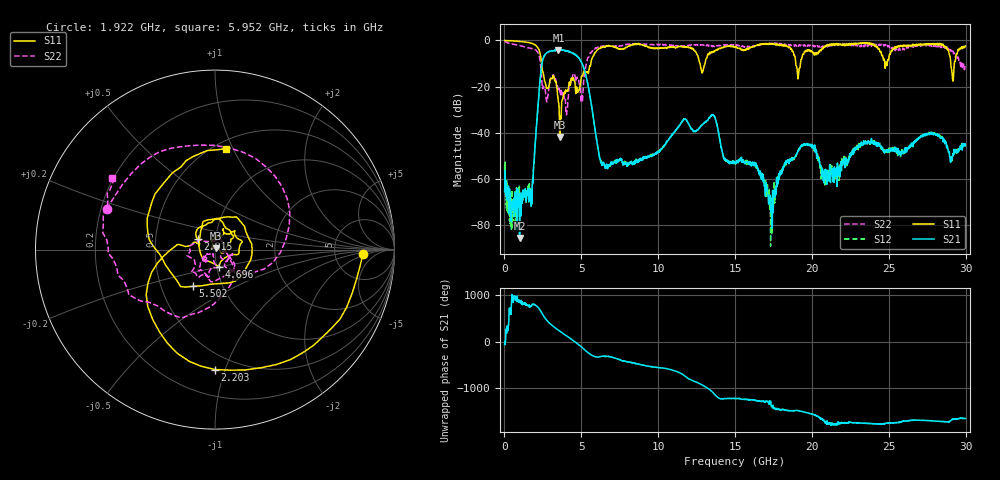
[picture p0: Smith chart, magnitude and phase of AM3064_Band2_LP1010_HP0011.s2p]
# Hz S DB R 50.0
!freq dBS11 angS11 dBS21 angS21 dBS12 angS12 dBS22 angS22
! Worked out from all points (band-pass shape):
!   1600 points, 10 MHz to 29.98 GHz, reference 50 ohm
!   highest |S21| = -4.09 dB at 3.515 GHz (marker M1); lowest = -85.6 dB at 984.7 MHz (marker M2)
!   |S21| within 3 dB of the highest: 2.559 GHz to 4.757 GHz (2.198 GHz wide, 60.1 % of centre)
!   lowest |S11| = -41.8 dB at 3.59 GHz (marker M3), VSWR 1.02, Z = 50.4 + j0.708 ohm
!   |S11| at or under -10 dB: 2.415 GHz to 5.619 GHz (3.205 GHz wide, 79.8 % of centre); 12.71 GHz to 13.05 GHz (330.9 MHz wide, 2.57 % of centre); 18.95 GHz to 19.25 GHz (304 MHz wide, 1.59 % of centre)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
!   |S22| runs from -32.2 to -0.3 dB; largest |S21 - S12| = 0.016
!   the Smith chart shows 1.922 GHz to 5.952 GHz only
!   S11 on the Smith chart (normalised r, x): 1.922 GHz: 10, -2; 2.203 GHz: 0.38, -0.92; 2.915 GHz: 0.82, +0.10; 4.696 GHz: 1.03, -0.20; 5.502 GHz: 0.72, -0.31; 5.952 GHz: 0.57, +0.94
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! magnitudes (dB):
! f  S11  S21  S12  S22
! 10 MHz  0.0  -65.5  -54.5  -0.3
! 328.6 MHz  -0.1  -64.3  -78.3  -1.3
! 984.7 MHz  -0.4  -85.6  -66.9  -2.2
! 1.922 GHz  -1.7  -52.5  -53.1  -3.8
! 2.203 GHz  -3.5  -26.4  -26.5  -5.5
! 2.915 GHz  -19.0  -4.8  -4.7  -19.1
! 3.515 GHz  -26.8  -4.1  -4.2  -21.8
! 3.59 GHz  -41.8  -4.2  -4.2  -21.9
! 4.696 GHz  -20.2  -6.7  -6.7  -16.0
! 5.015 GHz  -15.4  -9.5  -9.4  -24.5
! 5.502 GHz  -12.4  -21.7  -21.7  -7.0
! 5.952 GHz  -4.9  -40.9  -41.1  -3.2
! 6.664 GHz  -2.4  -53.8  -54.0  -2.4
! 10 GHz  -3.4  -48.1  -48.6  -1.9
! 13.54 GHz  -5.3  -32.2  -32.1  -2.6
! 15 GHz  -2.7  -53.3  -53.2  -1.9
! 17.37 GHz  -1.6  -71.9  -74.0  -1.2
! 19.99 GHz  -4.7  -45.7  -46.0  -2.0
! 20.89 GHz  -2.2  -55.8  -58.4  -2.8
! 25 GHz  -7.9  -47.3  -46.7  -2.3
! 29.18 GHz  -17.6  -49.8  -50.0  -4.8
! 29.98 GHz  -2.4  -45.6  -46.0  -10.3
